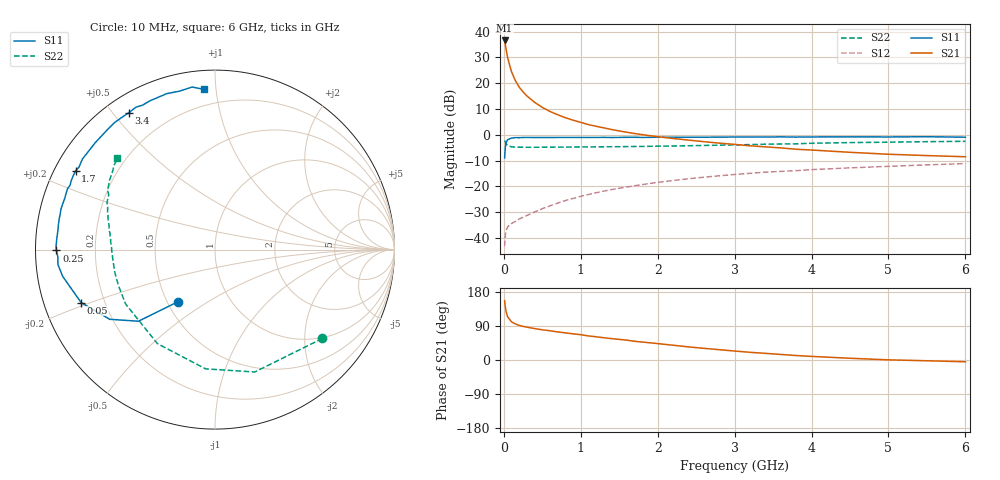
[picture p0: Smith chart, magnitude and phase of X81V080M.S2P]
! SIEMENS Small Signal Semiconductors
! BFP136W
! Si NPN RF Bipolar Junction Transistor in SOT343
! VCE = 1 V  IC = 80 mA
! Common Emitter S-Parameters:  September  1994
# GHz  S  MA  R  50
!  f  S11  S21  S12  S22
! GHz  MAG  ANG  MAG  ANG  MAG  ANG  MAG  ANG
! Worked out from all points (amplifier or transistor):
!   40 points, 10 MHz to 6 GHz, reference 50 ohm
!   highest |S21| = 36.6 dB at 10 MHz (marker M1)
!   |S21| within 3 dB of that: start of sweep to 27.12 MHz
!   unconditionally stable (mu >= 1): 458.2 MHz to 3.413 GHz; 3.714 GHz to 3.916 GHz; 5.863 GHz to end of sweep
!   at 200 MHz: K = 0.69, MSG = 25.6 dB, |S12| = -32.7 dB
!   at 1.5 GHz: K = 1.12, MAG = 9.0 dB, |S12| = -20.8 dB
!   at 6 GHz: K = 1.02, MAG = 0.5 dB, |S12| = -11.2 dB
!   S11 on the Smith chart (normalised r, x): 10 MHz: 0.57, -0.38; 50 MHz: 0.11, -0.19; 250 MHz: 0.06, -0.00; 1.7 GHz: 0.06, +0.26; 3.4 GHz: 0.07, +0.55; 6 GHz: 0.10, +0.93
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0.01  0.3555 -125.3  67.28 156.6  0.0069 65.7  0.7767 -39.6
0.02  0.5839 -136.9  55.38 138.6  0.0115 51.4  0.717 -72.0
0.03  0.7035 -146.5  44.81 126.9  0.0139 43.3  0.6665 -94.5
0.05  0.8022 -158.4  30.78 113.6  0.0164 34.2  0.6143 -121.5
0.1  0.8614 -170.0  16.57 100.7  0.019 33.2  0.583 -148.6
0.15  0.8789 -174.6  11.18 95.0  0.0208 36.0  0.5741 -159.1
0.2  0.8765 -177.4  8.376 91.4  0.0232 39.6  0.5724 -164.6
0.25  0.8838 -179.7  6.752 88.7  0.0251 42.9  0.5724 -168.1
0.3  0.886 178.8  5.641 86.7  0.0272 45.9  0.571 -170.6
0.4  0.8832 175.5  4.248 82.9  0.0318 50.5  0.5717 -173.8
0.5  0.8815 173.0  3.387 79.7  0.0368 54.4  0.5725 -176.1
0.6  0.8833 171.3  2.825 77.2  0.0418 56.3  0.5732 -177.7
0.7  0.8849 168.8  2.441 74.1  0.0472 58.3  0.575 -178.9
0.9  0.8873 165.4  1.915 69.0  0.0581 60.0  0.5767 178.7
1.1  0.8843 161.1  1.572 63.5  0.0693 60.5  0.5804 177.0
1.7  0.8921 150.6  1.054 49.4  0.1024 58.1  0.5909 171.8
2.2  0.8925 142.2  0.845 39.0  0.1294 54.2  0.6038 167.7
3.2  0.9012 125.3  0.61 20.3  0.1783 44.3  0.643 158.4
3.4  0.9012 122.3  0.582 17.5  0.188 42.1  0.6555 156.6
4.5  0.9096 107.2  0.456 4.6  0.2278 31.7  0.7036 146.6
5.5  0.9145 98.0  0.394 -2.0  0.2602 23.6  0.7335 139.9
6  0.8948 93.9  0.374 -4.7  0.276 19.3  0.7447 136.9
